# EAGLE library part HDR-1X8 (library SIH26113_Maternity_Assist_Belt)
1x8 2.54 mm pin header
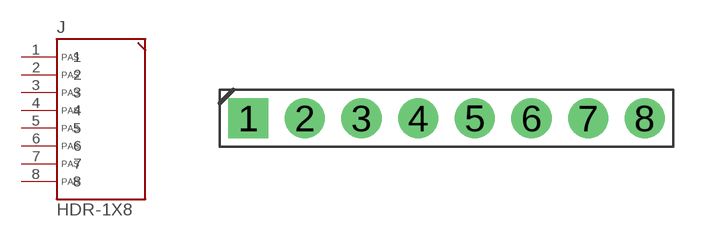
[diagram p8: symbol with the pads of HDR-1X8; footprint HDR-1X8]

Designator prefix J

## HDR-1X8  [HDR-1X8]
1  1  pas
2  2  pas
3  3  pas
4  4  pas
5  5  pas
6  6  pas
7  7  pas
8  8  pas

## Footprint HDR-1X8 (pad centres in mm)
1x8 2.54 mm through-hole pin header. Drill 1.0 mm / pad 1.8 mm suits the 0.64 mm square posts used by all common 2.54 mm headers. Pad 1 is square.
drill 1 pad 1.8 square: 1 -8.89,0
drill 1 pad 1.8: 2 -6.35,0; 3 -3.81,0; 4 -1.27,0; 5 1.27,0; 6 3.81,0; 7 6.35,0; 8 8.89,0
